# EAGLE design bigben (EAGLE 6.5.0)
AUTHOR: Brad Campbell; REV: A; TITLE: BigBen
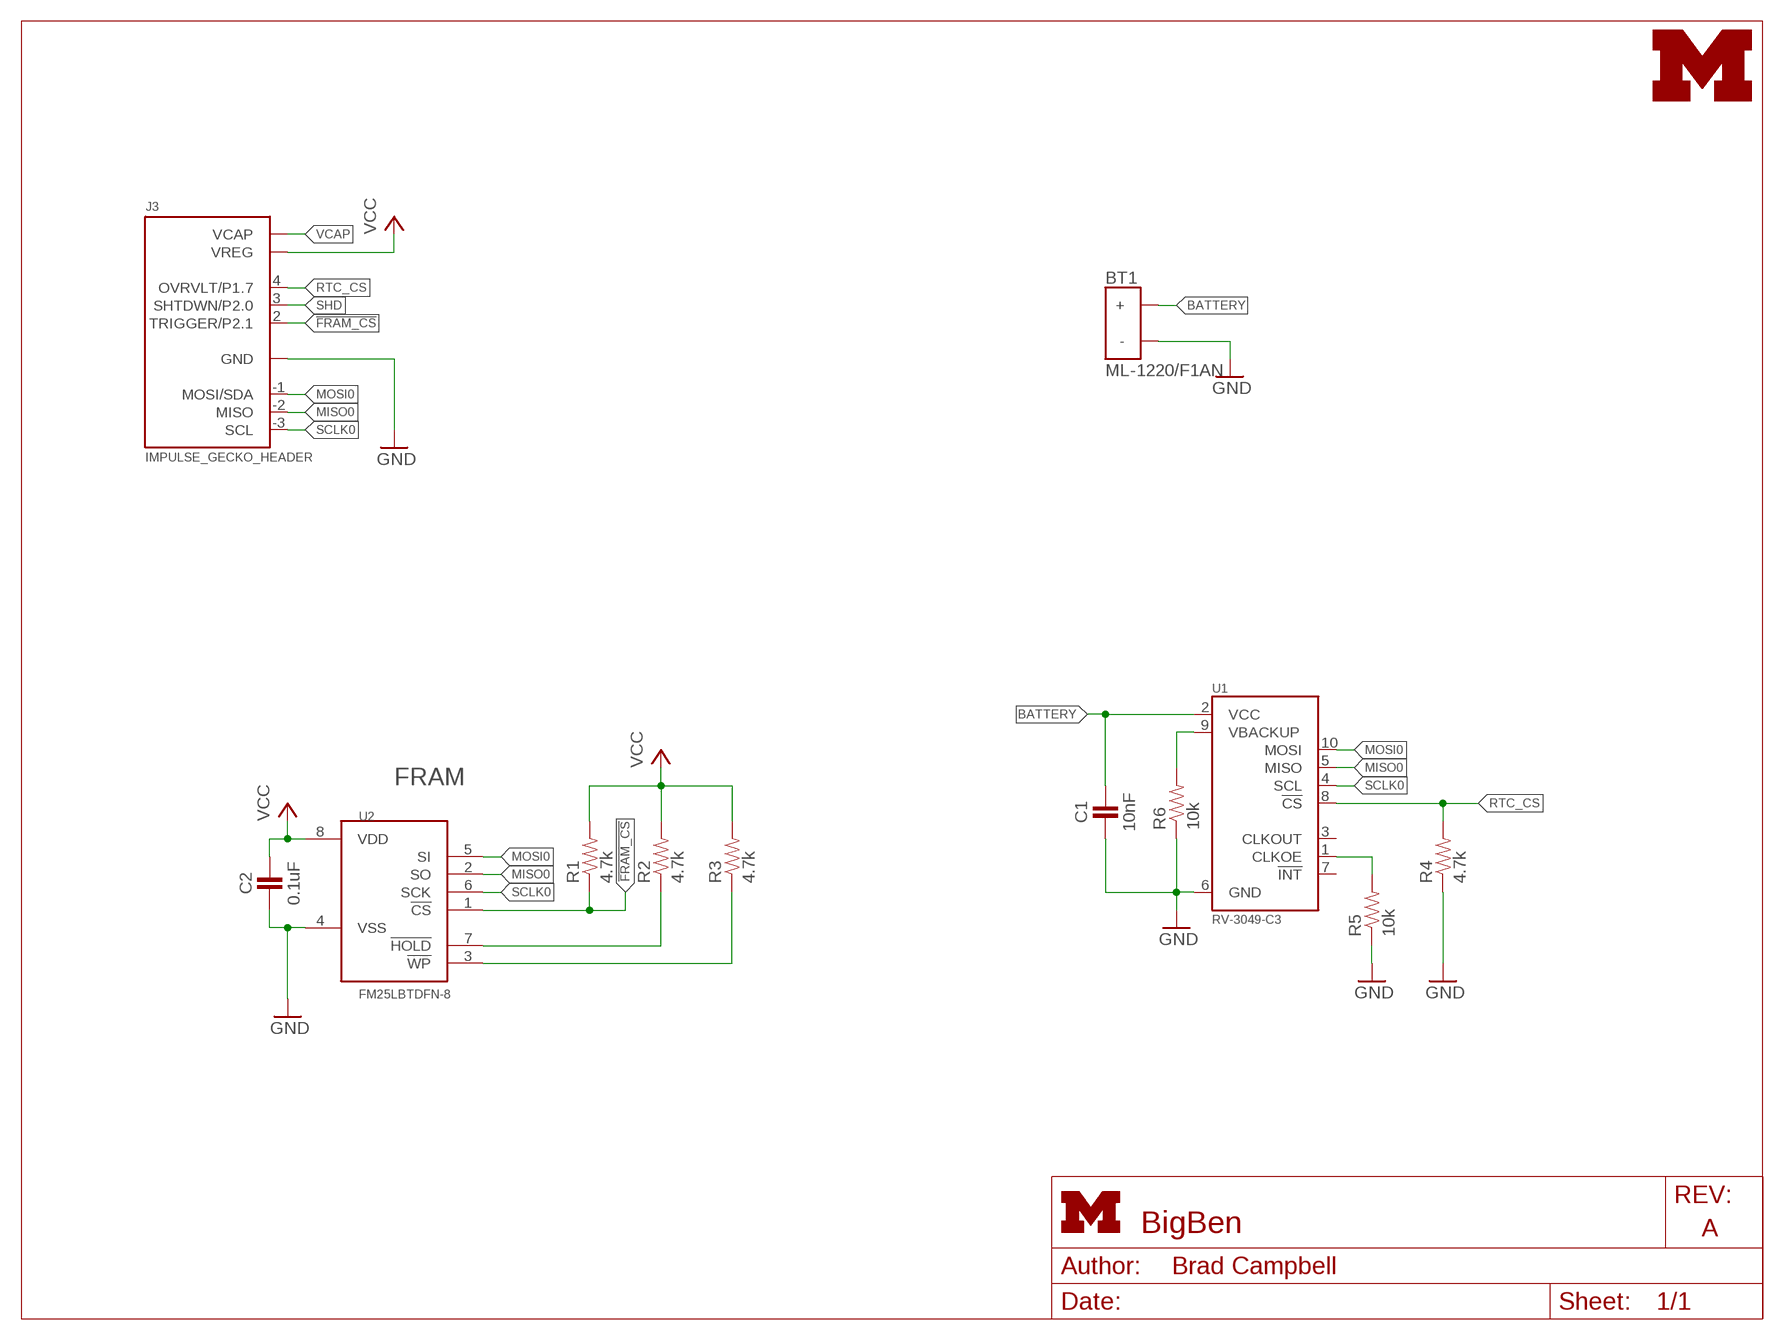
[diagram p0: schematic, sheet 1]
FRAME1 (LETTER_L): HEIGHT: 8.5in; WIDTH: 11in

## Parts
BT1  ML-1220/F1AN  [ML-1220/F1BN]
C1  10nF  CAPACITOR  [0402_CAP]
C2  0.1uF  CAPACITOR  [0402_CAP]
J3  IMPULSE_GECKO_HEADER  [HEADER1X9/0.05IN]
LOGO1  UMICH_SOLID_TINY  [UMICH_SOLID_50MIL]
R1  4.7k  RESISTOR  [0402_RES]
R2  4.7k  RESISTOR  [0402_RES]
R3  4.7k  RESISTOR  [0402_RES]
R4  4.7k  RESISTOR  [0402_RES]
R5  10k  RESISTOR  [0402_RES]
R6  10k  RESISTOR  [0402_RES]
U1  RV-3049-C3  [MICRO-CRYSTAL-C3]
U2  FM25LBTDFN-8  [TDFN-8]

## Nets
!FRAM_CS: J3.2(TRIGGER/P2.1) R1.1 U2.1(!CS)
!FRAM_HOLD: R2.1 U2.7(!HOLD)
!FRAM_WP: R3.1 U2.3(!WP)
BATTERY: BT1.POS(+) C1.1 U1.2(VCC)
GND: BT1.NEG(-) C1.2 C2.2 J3.0(GND) R4.1 R5.1 R6.1 U1.6(GND) U2.4(VSS)
MISO0: J3.-2(MISO) U1.5(MISO) U2.2(SO)
MOSI0: J3.-1(MOSI/SDA) U1.10(MOSI) U2.5(SI)
N$6: R6.2 U1.9(VBACKUP)
N$7: R5.2 U1.1(CLKOE)
RTC_CS: J3.4(OVRVLT/P1.7) R4.2 U1.8(!CS)
SCLK0: J3.-3(SCL) U1.4(SCL) U2.6(SCK)
SHD: J3.3(SHTDWN/P2.0)
VCAP: J3.5(VCAP)
VCC: C2.1 J3.1(VREG) R1.2 R2.2 R3.2 U2.8(VDD)
Unconnected: U1.3(CLKOUT) U1.7(!INT)

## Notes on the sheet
- FRAM

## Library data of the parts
BT1 = batteries:ML-1220/F1AN: BATTERY LITH 3V RECHARGE PC PINS; DIGIKEY: P663-nd; MOUSER: 658-ML-1220/F1BN
C1 C2 = passives:CAPACITOR: 0402 Capacitor
J3 = gecko:IMPULSE_GECKO_HEADER: Header on the impulse EPIC-esque board.
LOGO1 = logos:UMICH_SOLID
R1-R6 = passives:RESISTOR: Resistor
U1 = chips:RV-3049-C3: The RV-3049-C3 is an ultra miniature Real-Time-Clock Module with embedded Crystal. This RTC has an SPI Bus (4-wire Serial- Interface) and offers temperature compensated time.
U2 = chips:FM25LB: IC FRAM 4KBIT 10MHZ 8SOIC; MOUSER: 877-FM25V20-DG

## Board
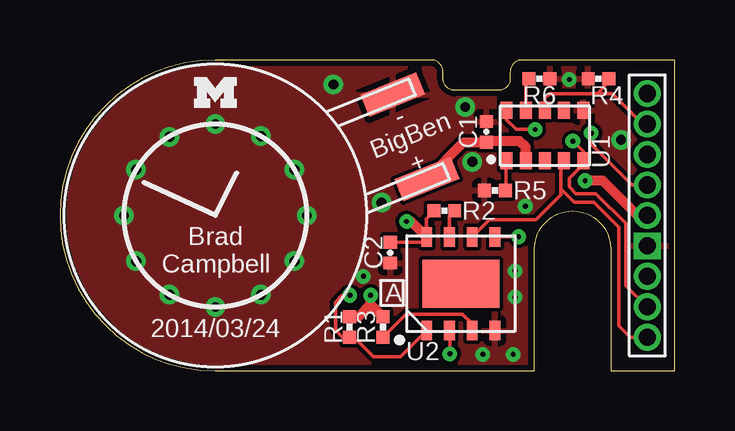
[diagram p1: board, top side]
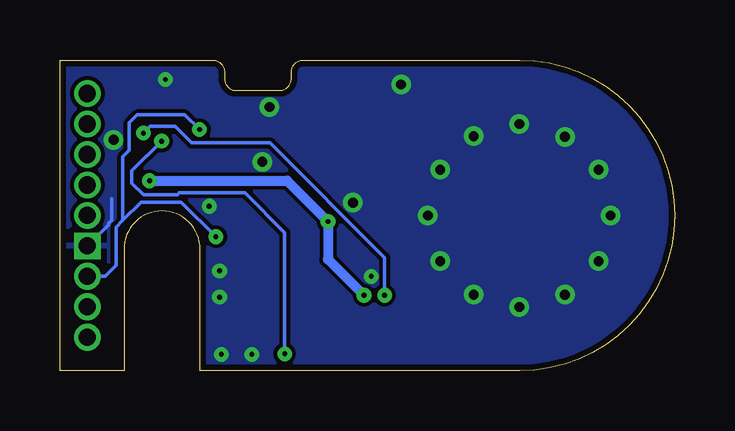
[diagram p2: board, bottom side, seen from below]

Size 25.63 x 12.95 mm. Coordinates in mm from the lower left corner, seen from the top.
Outline: 6.48,0 19.79,0 19.79,5.08 arc-180 22.96,5.08 22.96,0 25.63,0 25.63,12.95 19.28,12.95 arc90 18.77,12.45 18.77,12.19 arc-90 18.26,11.68 16.48,11.68 arc-90 15.98,12.19 15.98,12.45 arc90 15.47,12.95 6.48,12.95 arc180 6.48,0
Copper layers (1*16): Top 0.0178mm / dielectric 59mil / Bottom 0.0178mm
Design rules "sunstone-2lyr_v1.0.0.3 *": minimum track width 6mil, minimum drill 14mil, track to track 6mil, track to pad 6mil, pad to pad 6mil, via to via 6mil, smd to smd 6mil, copper to edge 10mil, drill to drill 16mil, minimum pad ring 8mil, minimum via ring 8mil, stop-mask expansion 3mil, vias tented up to drill 100mil, thermal gap 10mil

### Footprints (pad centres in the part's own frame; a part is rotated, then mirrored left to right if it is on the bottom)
ML-1220/F1BN = smd 2.5 x 1: NEG 8.75,1.9; POS 8.75,-1.9
0402_CAP = smd 0.536 x 0.546: 1 -0.433,0; 2 0.433,0
HEADER1X9/0.05IN = drill 0.711 pad 1.016 square: 0 -1.27,0 | drill 0.711 pad 1.016: 1 0,0; 2 1.27,0; 3 2.54,0; 4 3.81,0; 5 5.08,0; -1 -2.54,0; -2 -3.81,0; -3 -5.08,0
0402_RES = smd 0.536 x 0.546: 1 -0.433,0; 2 0.433,0
MICRO-CRYSTAL-C3 = smd 0.5 x 0.7: 1 -1.6,-1.05; 2 -0.8,-1.05; 3 0,-1.05; 4 0.8,-1.05; 5 1.6,-1.05; 6 1.6,1.05; 7 0.8,1.05; 8 0,1.05; 9 -0.8,1.05; 10 -1.6,1.05
TDFN-8 = smd 0.45 x 0.8: 1 -1.425,-1.95; 2 -0.475,-1.95; 3 0.475,-1.95; 4 1.425,-1.95; 5 1.425,1.95; 6 0.475,1.95; 7 -0.475,1.95; 8 -1.425,1.95 | smd 3.2 x 2: NC 0,0

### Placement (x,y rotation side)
BT1  6.48,6.48 22 top
C1  17.78,9.96 90 top
C2  13.77,4.93 270 top
J3  24.49,6.48 90 top
LOGO1  6.48,11.61 0 top
R1  12.06,1.83 90 top
R2  16.03,6.67 180 top
R3  13.46,1.83 90 top
R4  22.45,12.17 0 top
R5  18.14,7.52 0 top
R6  19.99,12.17 180 top
U1  20.22,9.8 0 top
U2  16.71,3.63 0 top

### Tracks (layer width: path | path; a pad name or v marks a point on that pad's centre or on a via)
!FRAM_CS  (via drill 0.2)
  Top 0.152: U2.1 14.19,0.58 13.08,0.58 12.45,1.22 R1.1 11.78,1.4 11.48,1.7 11.48,2.87 11.76,3.15 v12.09,3.15 | J3.2 23.85,7.75 22.15,9.45 v22.15,9.91
  Bottom 0.152: v22.15,9.91 21.87,10.19 20.83,10.19 20.14,9.5 16.87,9.5 12.09,4.72 v12.09,3.15
!FRAM_HOLD
  Top 0.152: U2.7 16.24,6.45 R2.1
!FRAM_WP
  Top 0.152: U2.3 17.19,1.96 16.79,2.36 14.43,2.36 R3.1
BATTERY
  Top 0.406: 17.8,9.5 C1.1 | U1.2 19.42,9.33 19.18,9.58 17.83,9.58 C1.1 | C1.1 16.83,9.52 BT1.POS
GND  (via drill 0.2, 0.41)
  Bottom 0.152: J3.0 23.6,6.1 23.6,6.15 23.47,6.27 23.47,7.16
  other vias: 11.4,11.94 17.2,8.71 23.39,9.63 19.41,6.86 21.23,12.14 18.97,4.17 18.97,3.07 12.65,3.94 13.41,7.01 16.89,11 18.9,0.69 17.63,0.69 6.48,10.29 6.48,2.67 10.29,6.48 2.67,6.48 9.78,8.38 8.38,9.78 4.57,3.17 3.18,4.57 3.18,8.38 8.38,3.17 4.57,9.75 9.78,4.57
  pour Top: 26.14,13.72 26.14,-0.51 -1.37,-0.51 -1.37,13.72
  pour Bottom: -1.35,13.72 26.14,13.72 26.14,-0.51 -1.35,-0.51
MISO0  (via drill 0.2)
  Top 0.152: J3.-2 23.6,3.56 23.6,6.15 22.35,7.39 21.51,7.39 21.23,7.67 21.23,8.03 21.82,8.61 U1.5 21.82,9.14 v21.39,9.58 | v16.26,0.71 16.26,1.66 U2.2
  Bottom 0.152: v16.26,0.71 16.26,5.77 17.91,7.42 20.65,7.42 20.73,7.34 22.15,7.34 22.63,7.82 22.63,8.33 v21.39,9.58
MOSI0  (via drill 0.2)
  Top 0.152: v19.13,5.59 U2.5 | U1.10 18.62,10.46 19.02,10.06 v19.81,10.06
  Bottom 0.152: J3.-1 23.75,3.94 23.29,4.39 23.29,5.99 23.01,6.27 | v19.13,5.59 20.57,7.04 22.25,7.04 23.01,6.27 | v19.81,10.06 20.42,10.67 22.4,10.67 22.73,10.34 22.73,9.2 23.01,8.91 23.01,6.27
N$6
  Top 0.152: U1.9 19.42,12.03 R6.2
N$7
  Top 0.152: U1.1 18.59,8.73 18.59,7.54 R5.2
RTC_CS
  Top 0.152: U1.8 20.22,11.35 20.42,11.56 22.4,11.56 | 22.4,11.56 22.89,12.04 R4.2 | J3.4 24.31,10.29 23.04,11.56 22.4,11.56
SCLK0
  Top 0.152: J3.-3 23.77,1.4 23.29,1.88 23.29,5.99 22.25,7.04 21.44,7.04 20.88,7.59 | U2.6 17.9,6.3 19.84,6.3 20.88,7.34 20.88,7.59 | 20.88,7.59 20.88,8.62 U1.4
VCC  (via drill 0.2)
  Top 0.152: R2.2 15.61,6.67 15.29,6.35 U2.8 15.07,5.36 C2.1
  Top 0.406: v14.45,6.22 14.65,6.22 U2.8 | 12.95,2.77 R3.2 | 12.95,2.77 v12.95,3.15 | J3.1 24.08,6.48 22.63,7.92 v21.89,7.92 | 12.95,2.77 12.45,2.26 R1.2
  Bottom 0.406: v12.95,3.15 14.45,4.65 v14.45,6.22 16.15,7.92 v21.89,7.92

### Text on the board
tPlace: - | BigBen | + | Brad / Campbell | A | 2014/03/24
tDocu: VCAP | OV | SHTD | TRIG | VREG | GND | MOSI | MISO | SCL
